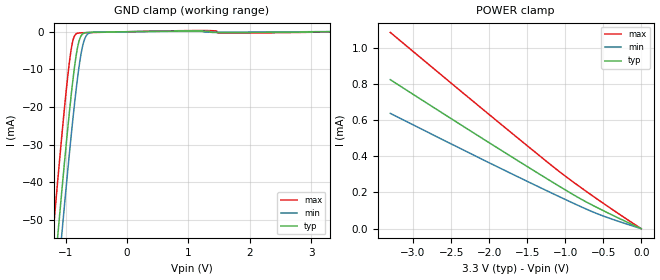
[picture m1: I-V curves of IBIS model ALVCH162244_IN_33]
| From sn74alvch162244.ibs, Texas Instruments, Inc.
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[Model]   ALVCH162244_IN_33
Model_type  Input
Vinl=0.8
Vinh=2.0
| variable   typ   min   max
C_comp   5.09pF   3.97pF   6.29pF
[Temperature Range]   40   100   -40
| Ambient temperature   25   85   -40
[Voltage range]   3.3   3   3.6
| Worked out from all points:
|   GND clamp passes 1 mA (typ) near -0.75 V on its own axis
[GND Clamp]
| ALVCH162244_IN_33
|   Voltage   I(typ)   I(min)   I(max)
-3.3V     -478.4mA   -488.5mA   -465.8mA
-1.215V   -69.67mA   -81.15mA   -54.95mA
-1.185V   -64.11mA   -75.6mA    -49.36mA
-1.125V   -53.11mA   -64.6mA    -38.36mA
-1.065V   -42.34mA   -53.78mA   -27.68mA
-925mV    -18.84mA   -29.68mA   -6.119mA
-875mV    -11.59mA   -21.76mA   -1.826mA
-820mV    -5.223mA   -13.82mA   -467uA
-770mV    -1.782mA   -7.754mA   -308.8uA
-715mV    -476.7uA   -3.107mA   -272.7uA
-585mV    -155.7uA   -204.3uA   -219.8uA
3.3V      8.676pA    40.66uA    -79.23uA
[POWER Clamp]
| ALVCH162244_IN_33
|   Voltage   I(typ)   I(min)   I(max)
-3.3V     822.6uA    636.7uA    1.084mA
-1.98V    469.3uA    359.8uA    623.3uA
-1.075V   233.5uA    176.2uA    314.6uA
-795mV    164uA      121.7uA    227.5uA
-565mV    113.3uA    80.24uA    159.3uA
-48.03fV  8.677pA    12.17pA    9.125pA
